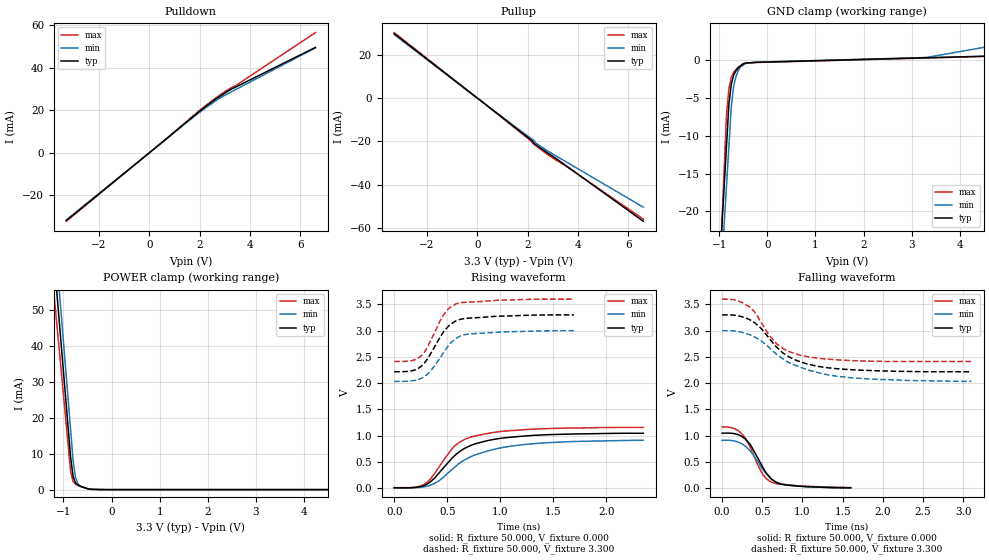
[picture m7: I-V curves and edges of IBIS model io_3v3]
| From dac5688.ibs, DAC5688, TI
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[Model]   io_3v3
Model_type I/O
Vinl = 1.00000V
Vinh = 2.30000V
Vref=0.000E+00
Rref=1.000E+06
Cref=0.000E+00
Vmeas=1.650E+00
C_comp   5.910E-13   5.910E-13   5.910E-13
[Voltage Range]   3.300E+00   3.000E+00   3.600E+00
[POWER Clamp Reference]   3.300E+00   3.000E+00   3.600E+00
[GND Clamp Reference]   0.000E+00   0.000E+00   0.000E+00
[Pullup Reference]   3.300E+00   3.000E+00   3.600E+00
[Pulldown Reference]   0.000E+00   0.000E+00   0.000E+00
[Temperature Range]   25   85   -40
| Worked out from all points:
|   slope of the pulldown table from 0 to 0.495 V, typ, clamps not added: 103 ohm
|   slope of the pullup table from 0 to 0.495 V, typ, clamps not added: 112 ohm
|   GND clamp passes 1 mA (typ) near -0.60 V on its own axis
|   POWER clamp passes 1 mA (typ) near -0.66 V on its own axis
|   rising waveform, R_fixture 50.000, V_fixture 0.000: 20-80 % time 364ps typ, 475ps min, 297ps max; typ from 0.009 V to 1.05 V
|   falling waveform, R_fixture 50.000, V_fixture 0.000: 20-80 % time 245ps typ, 267ps min, 220ps max; typ from 1.05 V to 0.007 V
|   rising waveform, R_fixture 50.000, V_fixture 3.300: 20-80 % time 206ps typ, 217ps min, 186ps max; typ from 2.22 V to 3.3 V
|   falling waveform, R_fixture 50.000, V_fixture 3.300: 20-80 % time 468ps typ, 644ps min, 369ps max; typ from 3.3 V to 2.22 V
[GND Clamp]
-3.3V     -282mA     -274.9mA   -377.7mA
-850mV    -11.37mA   -16.68mA   -7.237mA
-800mV    -5.853mA   -11.41mA   -3.796mA
-750mV    -3.202mA   -6.143mA   -2.294mA
-700mV    -1.976mA   -3.437mA   -1.607mA
-650mV    -1.4mA     -2.132mA   -1.255mA
-600mV    -1.005mA   -1.343mA   -902.4uA
-500mV    -522.7uA   -676.6uA   -484.6uA
-450mV    -404.4uA   -454.6uA   -456uA
-225mV    -312.6uA   -291uA     -337.5uA
3.3V      290.5uA    320.4uA    253.4uA
6.6V      855.2uA    3.995mA    806.5uA
[POWER Clamp]
-3.3V     401.5mA    420.6mA    355.3mA
-1.15V    56.98mA    65.99mA    47.91mA
-1.1V     48.96mA    57.74mA    40.76mA
-1.05V    40.95mA    49.49mA    33.61mA
-850mV    8.898mA    16.5mA     5.012mA
-800mV    3.735mA    8.256mA    2.309mA
-750mV    1.885mA    3.473mA    1.533mA
-700mV    1.287mA    1.638mA    1.167mA
-650mV    955.1uA    913.3uA    892.3uA
-450mV    115.2uA    77.27uA    93.22uA
-225mV    0A         0A         37.29uA
6.6V      0A         0A         0A
[Pullup]
-3.3V     29.65mA    29.26mA    30.17mA
800mV     -7.21mA    -7.042mA   -7.309mA
2.12V     -19.11mA   -18.46mA   -19.66mA
2.26V     -20.9mA    -19.71mA   -21.42mA
2.48V     -22.81mA   -21.96mA   -23.38mA
3.14V     -27.92mA   -26.72mA   -28.66mA
3.46V     -30.59mA   -28.9mA    -30.86mA
6.6V      -56.78mA   -50.29mA   -55.79mA
[Pulldown]
-3.3V     -31.83mA   -31.54mA   -32.18mA
1.46V     14.3mA     14.02mA    14.53mA
2.54V     24.43mA    23.62mA    24.88mA
3.26V     29.92mA    28.65mA    30.56mA
3.54V     31.55mA    30.38mA    32.42mA
6.6V      49.51mA    49.32mA    56.48mA
[Rising Waveform]
R_fixture = 50.000
V_fixture = 0.000
V_fixture_min = 0.000
V_fixture_max = 0.000
|  time   V(typ)   V(min)   V(max)
0s        9.179mV    8.47mV     9.998mV
190ps     13.44mV    9.915mV    17.87mV
285ps     52.82mV    27.02mV    74.48mV
340ps     119.9mV    55.54mV    171.2mV
425ps     294.1mV    143.6mV    411mV
565ps     610mV      390.8mV    795.6mV
750ps     835.4mV    624.5mV    989.1mV
995ps     947.6mV    763.9mV    1.078V
1.285ns   1.002V     842.5mV    1.122V
2.35ns    1.046V     913.6mV    1.158V
[Falling Waveform]
R_fixture = 50.000
V_fixture = 0.000
V_fixture_min = 0.000
V_fixture_max = 0.000
|  time   V(typ)   V(min)   V(max)
0s        1.048V     913.6mV    1.164V
175ps     1.031V     890.6mV    1.118V
290ps     936.1mV    800.3mV    951mV
360ps     806.5mV    687.4mV    745.7mV
445ps     572.8mV    503.2mV    437.3mV
500ps     414.8mV    371.6mV    280.2mV
610ps     181mV      175.9mV    117.2mV
695ps     96.06mV    105.7mV    81.52mV
820ps     56.15mV    61.27mV    64.42mV
1.6ns     6.653mV    8.47mV     14.82mV
[Rising Waveform]
R_fixture = 50.000
V_fixture = 3.300
V_fixture_min = 3.000
V_fixture_max = 3.600
|  time   V(typ)   V(min)   V(max)
0s        2.218V     2.034V     2.413V
170ps     2.237V     2.046V     2.43V
250ps     2.314V     2.087V     2.513V
300ps     2.421V     2.146V     2.636V
335ps     2.53V      2.215V     2.774V
470ps     2.991V     2.596V     3.312V
520ps     3.102V     2.737V     3.431V
585ps     3.191V     2.855V     3.511V
745ps     3.244V     2.942V     3.546V
1.695ns   3.3V       3V         3.6V
[Falling Waveform]
R_fixture = 50.000
V_fixture = 3.300
V_fixture_min = 3.000
V_fixture_max = 3.600
|  time   V(typ)   V(min)   V(max)
0s        3.3V       3V         3.6V
190ps     3.286V     2.985V     3.569V
370ps     3.186V     2.906V     3.413V
475ps     3.058V     2.817V     3.188V
575ps     2.874V     2.694V     2.934V
675ps     2.69V      2.55V      2.753V
815ps     2.516V     2.406V     2.613V
985ps     2.401V     2.296V     2.528V
1.58ns    2.258V     2.106V     2.432V
3.1ns     2.218V     2.034V     2.413V
[Ramp]
dV/dt_r   6.2470E-01/3.6246E-10   5.4256E-01/4.7377E-10   6.8962E-01/2.9559E-10
dV/dt_f   6.4939E-01/4.6635E-10   5.7979E-01/6.4223E-10   7.1207E-01/3.6728E-10
R_load = 50
